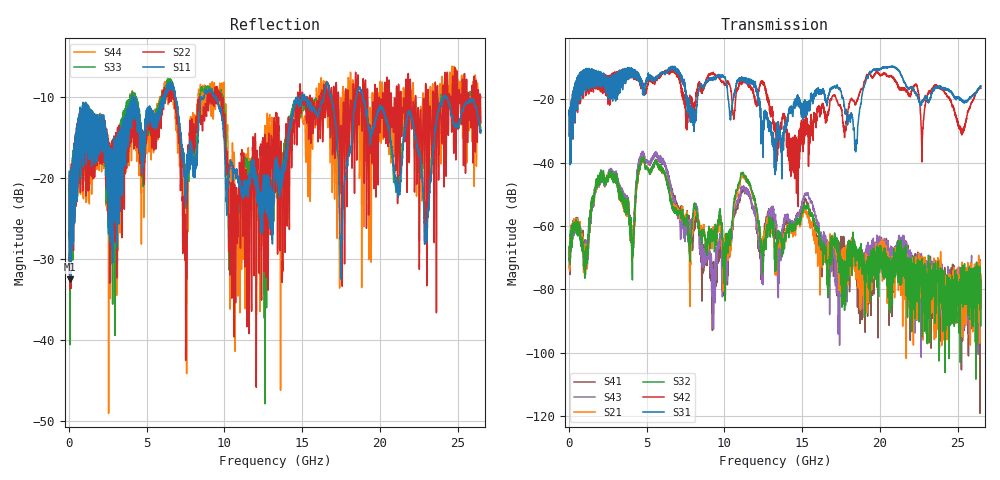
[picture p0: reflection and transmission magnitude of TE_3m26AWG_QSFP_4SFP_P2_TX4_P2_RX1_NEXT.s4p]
!Agilent Technologies,N5222A,MY51421691,A.10.00.00
!Agilent N5222A: A.10.00.00
!Date: Friday, January 30, 2015 12:35:21
!Correction: S11(Full 4 Port(1,2,3,4))
!S12(Full 4 Port(1,2,3,4))
!S13(Full 4 Port(1,2,3,4))
!S14(Full 4 Port(1,2,3,4))
!S21(Full 4 Port(1,2,3,4))
!S22(Full 4 Port(1,2,3,4))
!S23(Full 4 Port(1,2,3,4))
!S24(Full 4 Port(1,2,3,4))
!S31(Full 4 Port(1,2,3,4))
!S32(Full 4 Port(1,2,3,4))
!S33(Full 4 Port(1,2,3,4))
!S34(Full 4 Port(1,2,3,4))
!S41(Full 4 Port(1,2,3,4))
!S42(Full 4 Port(1,2,3,4))
!S43(Full 4 Port(1,2,3,4))
!S44(Full 4 Port(1,2,3,4))
!S4P File: Measurements: <S11,S12,S13,S14>,
!<S21,S22,S23,S24>,
!<S31,S32,S33,S34>,
!<S41,S42,S43,S44>:
# Hz S  dB  R 50.0
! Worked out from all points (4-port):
!   2650 points, 10 MHz to 26.5 GHz, reference 50 ohm
!   strongest paths, dB at 10 MHz, 6.63 GHz, 13.26 GHz, 19.88 GHz, 26.5 GHz:
!     S31: -25.0, -10.5, -43.8, -10.4, -15.7
!     S42: -24.8, -11.5, -27.7, -11.5, -16.5
!     S32: -66.5, -54.5, -74.4, -68.7, -77.1
!     S21: -69.6, -53.6, -73.2, -69.3, -86.0
!     S43: -73.2, -50.0, -58.8, -66.2, -76.9
!     S41: -69.3, -50.0, -62.6, -95.3, -81.3
!   lowest |S11| = -32.5 dB at 70 MHz (marker M1), VSWR 1.05, Z = 52.4 + j0.248 ohm
!   |S11| at or under -10 dB: start of sweep to 4.075 GHz; 9.453 GHz to 14.73 GHz (5.277 GHz wide, 43.6 % of centre); 18.91 GHz to 24.13 GHz (5.222 GHz wide, 24.3 % of centre)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
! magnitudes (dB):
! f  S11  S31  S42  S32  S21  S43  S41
! 10 MHz  -19.2  -25.0  -24.8  -66.5  -69.6  -73.2  -69.3
! 70 MHz  -32.5  -40.7  -38.1  -68.7  -73.3  -72.6  -75.3
! 5.6 GHz  -13.7  -13.7  -12.7  -40.1  -40.2  -37.6  -37.8
! 9.31 GHz  -9.9  -13.1  -12.0  -61.7  -61.0  -85.8  -75.6
! 11.17 GHz  -21.9  -13.9  -14.7  -43.4  -44.1  -47.8  -48.9
! 14.32 GHz  -12.4  -24.0  -42.6  -60.0  -62.2  -60.4  -61.1
! 26.5 GHz  -14.2  -15.7  -16.5  -77.1  -86.0  -76.9  -81.3
